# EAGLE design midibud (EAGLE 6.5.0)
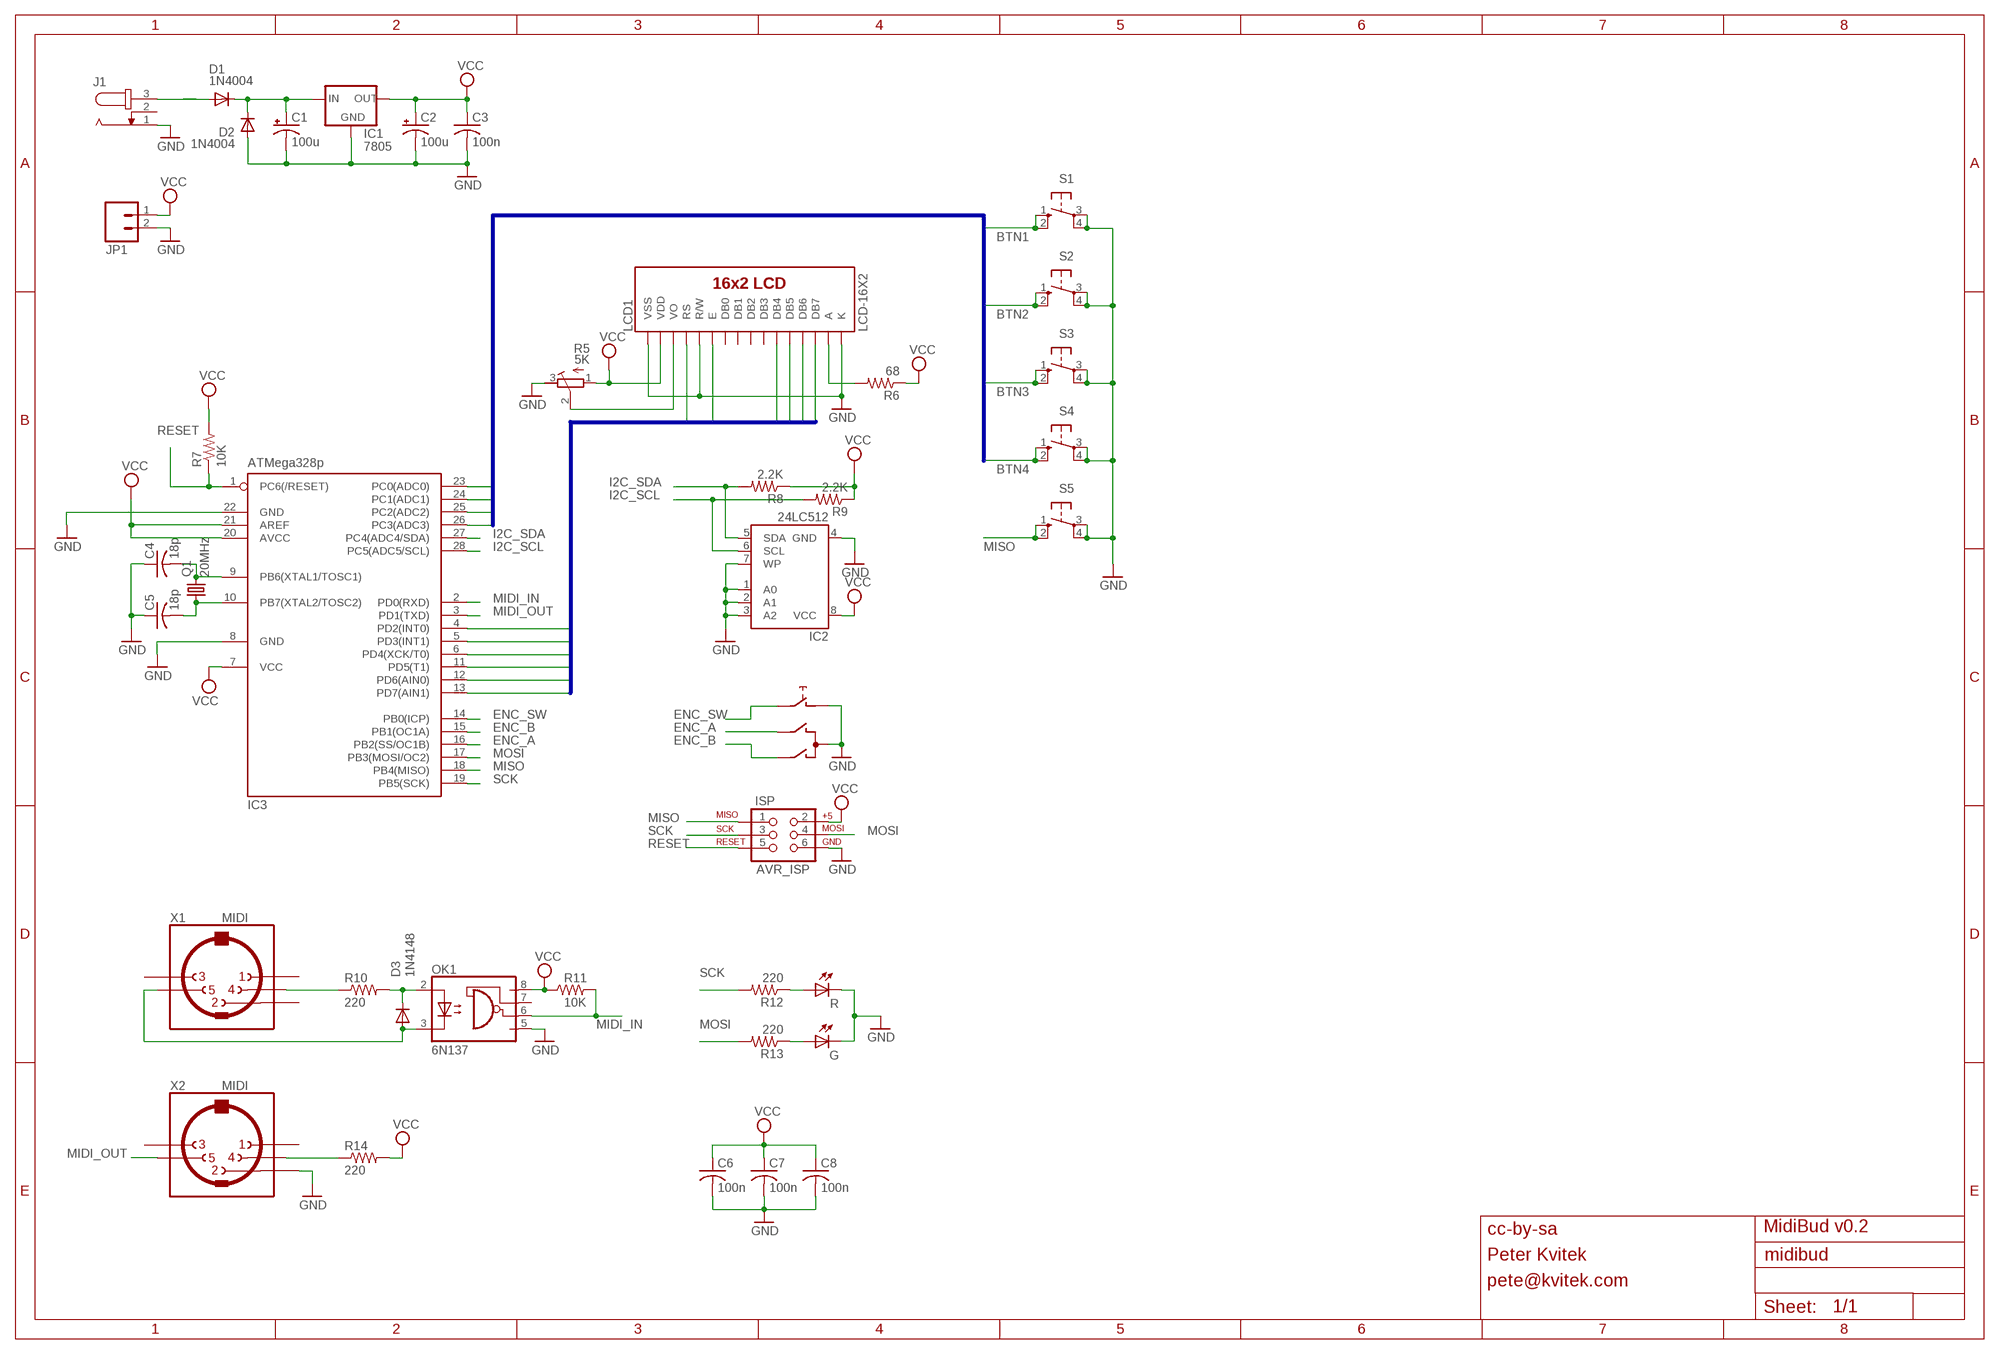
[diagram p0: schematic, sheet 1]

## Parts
C1  100u  CPOL-USE2.5-7  [E2,5-7]
C2  100u  CPOL-USE2.5-7  [E2,5-7]
C3  100n  C-US025-025X050  [C025-025X050]
C4  18p  C-US025-024X044  [C025-024X044]
C5  18p  C-US025-024X044  [C025-024X044]
C6  100n  C-US025-025X050  [C025-025X050]
C7  100n  C-US025-025X050  [C025-025X050]
C8  100n  C-US025-025X050  [C025-025X050]
D1  1N4004  [DO41-10]
D2  1N4004  [DO41-10]
D3  1N4148  DIODE-D-5  [D-5]
ENC1  Encoder  EC12E_SW  [ALPS_EC12E_SW]
G  LED3MM  [LED3MM]
IC1  7805  V_REG_78XXSIDE  [78XXL]
IC2  24LC512  AT24CP  [DIL08]
IC3  ATMega328p  MEGA8-P  [DIL28-3]
ISP  AVR_ISP  AVR_SPI_PRG_6PTH  [2X3]
J1  JACK-PLUG  [SPC4078_LARGER_HOLES]
JP1  M02  [1X02_LONGPADS]
LCD1  LCD-16X2  [LCD-16X2]
OK1  6N137  [DIL08]
Q1  20MHz  CRYSTALHC49U-V  [HC49U-V]
R  LED3MM  [LED3MM]
R5  5K  R-TRIMM3296P  [RTRIM3296P]
R6  68  R-US_0204/7  [0204/7]
R7  10K  R-US_0204/7  [0204/7]
R8  2.2K  R-US_0204/7  [0204/7]
R9  2.2K  R-US_0204/7  [0204/7]
R10  220  R-US_0204/7  [0204/7]
R11  10K  R-US_0204/7  [0204/7]
R12  220  R-US_0204/7  [0204/7]
R13  220  R-US_0204/7  [0204/7]
R14  220  R-US_0204/7  [0204/7]
S1  40-XX  [B3F-40XX]
S2  40-XX  [B3F-40XX]
S3  40-XX  [B3F-40XX]
S4  40-XX  [B3F-40XX]
S5  40-XX  [B3F-40XX]
X1  MIDI  MAB5SH  [MAB5SH]
X2  MIDI  MAB5SH  [MAB5SH]

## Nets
BTN1: IC3.23(PC0(ADC0)) S1.1(S) S1.2(S1)
BTN2: IC3.24(PC1(ADC1)) S2.1(S) S2.2(S1)
BTN3: IC3.25(PC2(ADC2)) S3.1(S) S3.2(S1)
BTN4: IC3.26(PC3(ADC3)) S4.1(S) S4.2(S1)
ENC_A: ENC1.B IC3.16(PB2(SS/OC1B))
ENC_B: ENC1.A IC3.15(PB1(OC1A))
ENC_SW: ENC1.E IC3.14(PB0(ICP))
GND: C1.- C2.- C3.2 C4.1 C5.1 C6.2 C7.2 C8.2 D2.A ENC1.C ENC1.D G.K(C) IC1.GND IC2.1(A0) IC2.2(A1) IC2.3(A2) IC2.4(GND) IC2.7(WP) IC3.8(GND) IC3.22(GND) ISP.6 J1.1 JP1.2 LCD1.1(VSS) LCD1.5(R/W) LCD1.16(K) OK1.5(GND) R5.3(E) R.K(C) S1.3(P) S1.4(P1) S2.3(P) S2.4(P1) S3.3(P) S3.4(P1) S4.3(P) S4.4(P1) S5.3(P) S5.4(P1) X2.2
I2C_SCL: IC2.6(SCL) IC3.28(PC5(ADC5/SCL)) R9.2
I2C_SDA: IC2.5(SDA) IC3.27(PC4(ADC4/SDA)) R8.2
LCD_DATA1: IC3.6(PD4(XCK/T0)) LCD1.11(DB4)
LCD_DATA2: IC3.11(PD5(T1)) LCD1.12(DB5)
LCD_DATA3: IC3.12(PD6(AIN0)) LCD1.13(DB6)
LCD_DATA4: IC3.13(PD7(AIN1)) LCD1.14(DB7)
LCD_EN: IC3.5(PD3(INT1)) LCD1.6(E)
LCD_RS: IC3.4(PD2(INT0)) LCD1.4(RS)
MIDI_IN: IC3.2(PD0(RXD)) OK1.6(VO) R11.2
MIDI_OUT: IC3.3(PD1(TXD)) X2.5
MISO: IC3.18(PB4(MISO)) ISP.1 S5.1(S) S5.2(S1)
MOSI: IC3.17(PB3(MOSI/OC2)) ISP.4 R13.2
N$2: D3.C OK1.2(A) R10.2
N$3: R14.1 X2.4
N$25: R12.1 R.A
N$26: G.A R13.1
N$72: R10.1 X1.4
N$73: D3.A OK1.3(C) X1.5
N$78: LCD1.3(VO) R5.2(S)
N$79: LCD1.15(A) R6.2
N$82: C5.2 IC3.10(PB7(XTAL2/TOSC2)) Q1.1
N$83: C4.2 IC3.9(PB6(XTAL1/TOSC1)) Q1.2
RESET: IC3.1(PC6(/RESET)) ISP.5 R7.1
SCK: IC3.19(PB5(SCK)) ISP.3 R12.2
VCC: C2.+ C3.1 C6.1 C7.1 C8.1 IC1.OUT IC2.8(VCC) IC3.7(VCC) IC3.20(AVCC) IC3.21(AREF) ISP.2 JP1.1 LCD1.2(VDD) OK1.8(VCC) R5.1(A) R6.1 R7.2 R8.1 R9.1 R11.1 R14.2
VPWR: D1.A J1.3
VREGIN: C1.+ D1.C D2.C IC1.IN
Unconnected: ENC1.GND1(G) ENC1.GND2(G) J1.2 LCD1.7(DB0) LCD1.8(DB1) LCD1.9(DB2) LCD1.10(DB3) OK1.7(VE) X1.1 X1.2 X1.3 X2.1 X2.3

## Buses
LCD_RS,LCD_EN,LCD_DATA[1..4]
BTN[1..4]

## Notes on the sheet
- cc-by-sa | MidiBud v0.2
- Peter Kvitek
- pete@kvitek.com

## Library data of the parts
C1 C2 = rcl:CPOL-US: POLARIZED CAPACITOR, American symbol
C3-C8 = rcl:C-US: CAPACITOR, American symbol
D1 D2 = diode:1N4004: DIODE
D3 = diode:DIODE-: DIODE
ENC1 = switch-alps:EC12E_SW: ALPS rotary Encoder EC12E series with switch
G R = led:LED: LED
IC1 = SparkFun:V_REG_78XX: Voltage Regulator Standard 7805 5V regulator. IGO (Input Ground Output). Spark Fun Electronics SKU : COM-00107
IC2 = atmel:AT24C*: 2-wire serial EEPROM
IC3 = atmel:MEGA8-P: MICROCONTROLLER 8 Kbytes FLASH, 1 kbytes SRAM, 512 bytes EEPROM, USART, 4-channel 10 bit ADC, 2-channel 8 bit ADC Pin compatible with Atmega48, ATMega88, ATMega168 Source: avr.lbr; OC_FARNELL: unknown; OC_NEWARK: unknown
ISP = SparkFun:AVR_SPI_PRG_6: AVR ISP 6 Pin This is the reduced ISP connector for AVR programming. Common on Arduino. This footprint will take up less PCB space and can be used with a 10-pin to 6-pin adapter such as SKU: BOB-08508
J1 = con-jack2:JACK-PLUG: DC POWER JACK Power Jack, DC, Right Angle, Through Hole, Rated 5A at 16VDC, PC Terminals Distributor: Farnell (www.Farnell.de) Drawing: 84N1161.pdf / 84N1162.pdf Manufacturer: SPC Technology (www.spctechnology.com) Type: SPC4077 / SPC 4078
JP1 = SparkFun:M02: Header 2
LCD1 = SparkFun:LCD-16X2
OK1 = kvitekp:6N137: MOTOROLA OPTO COUPLER; MPN: 6N137; OC_FARNELL: 1328376; OC_NEWARK: 52M1895
Q1 = crystal:CRYSTAL: CRYSTAL; OC_FARNELL: 1666969; OC_NEWARK: unknown
R5 = rcl:R-TRIMM: Trimm resistor
R6-R14 = rcl:R-US_: RESISTOR, American symbol
S1-S5 = og-switch:40-XX: OMRON SWITCH
X1 X2 = og-midi:MAB5SH: Female CONNECTOR 5 pins 90 deg. with shield, horizontal (DIN 41524)

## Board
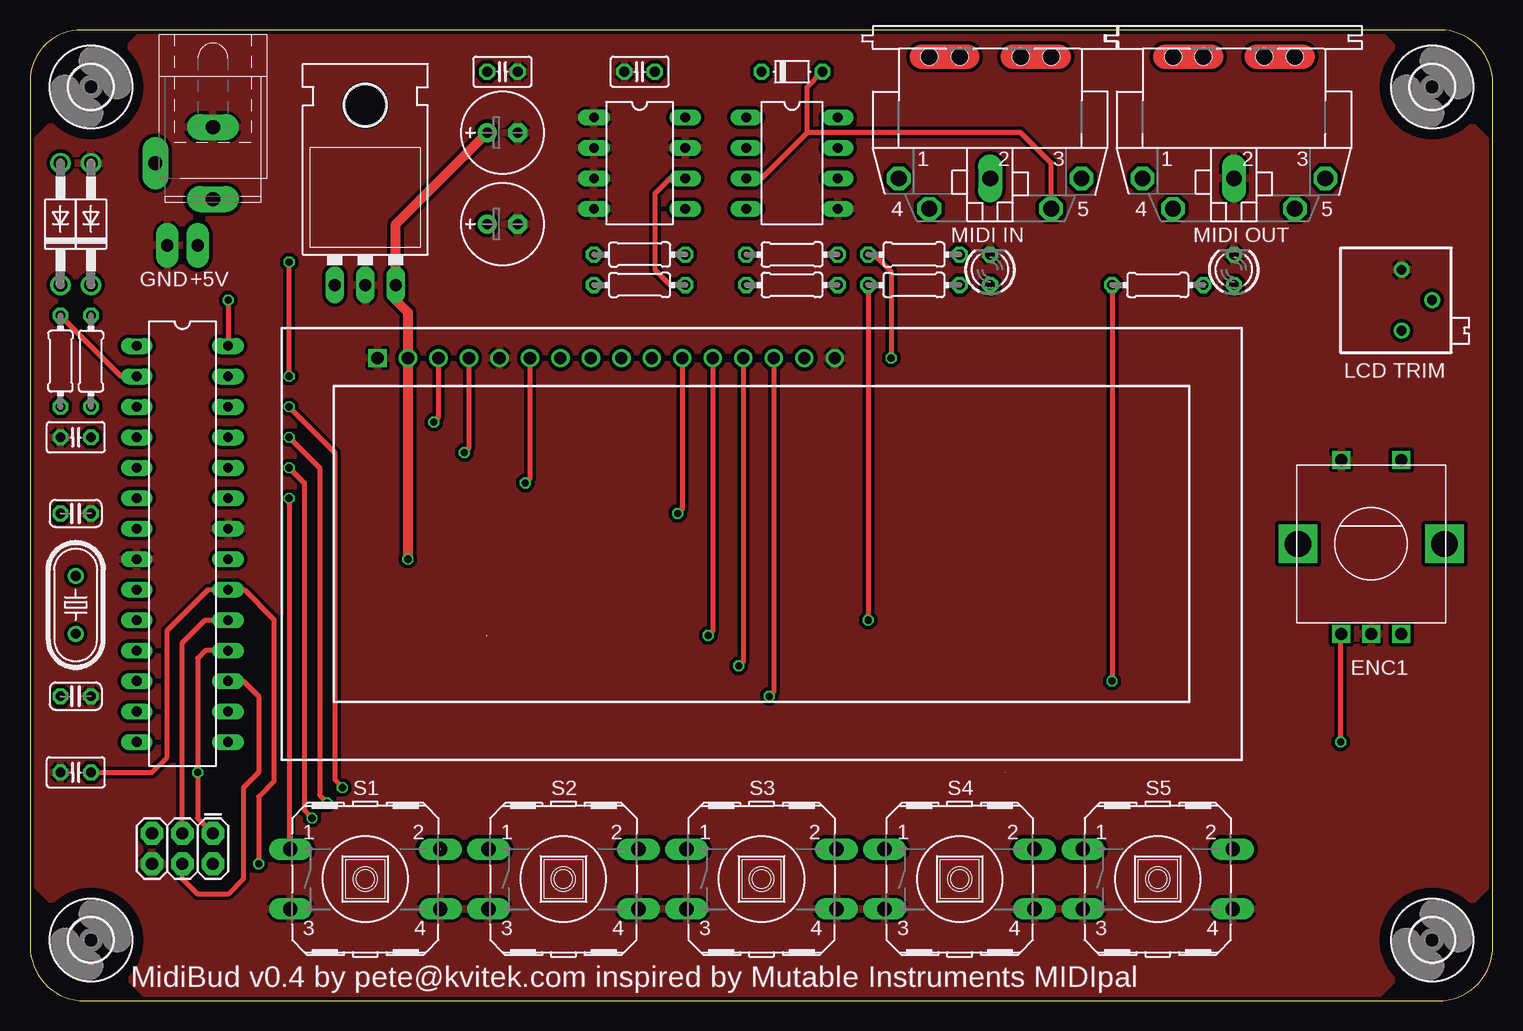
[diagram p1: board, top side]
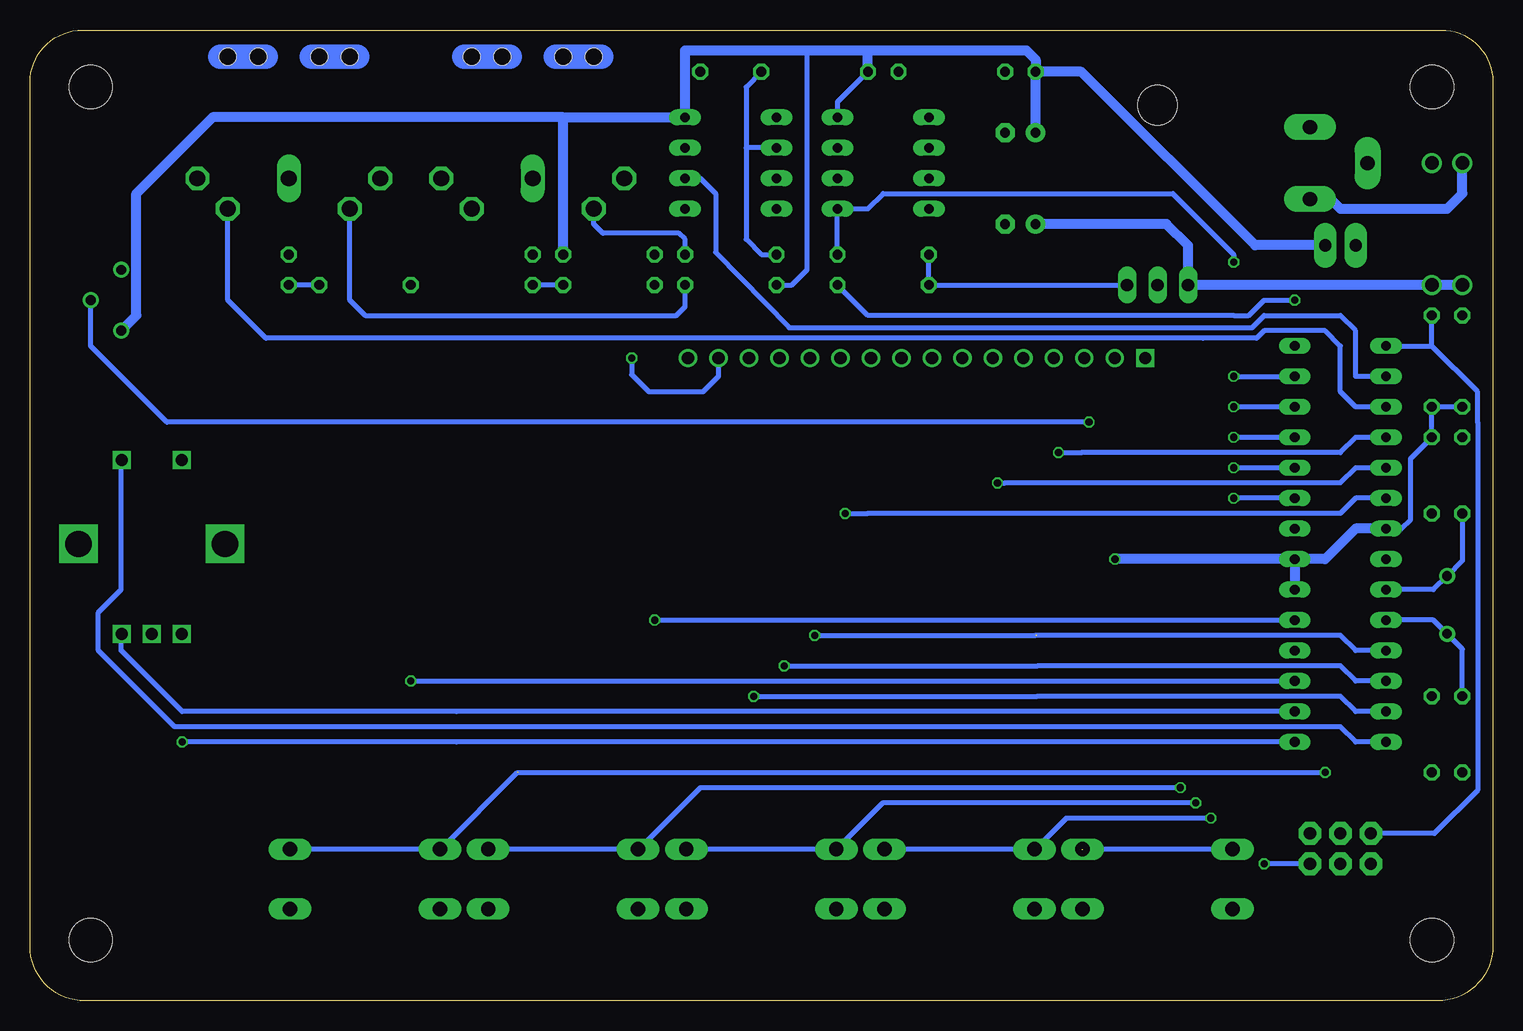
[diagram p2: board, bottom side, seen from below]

Size 121.9 x 80.95 mm. Coordinates in mm from the lower left corner, seen from the top.
Outline: 4.58,0 117.34,0 arc90 121.9,4.56 121.9,76.56 arc90 117.51,80.95 4.31,80.95 arc90 0,76.64 0,4.58 arc90 4.58,0
Copper layers (1*16): Top 0.035mm / dielectric 1.5mm / Bottom 0.035mm
Design rules "default": minimum track width 8mil, minimum drill 16mil, track to track 8mil, track to pad 8mil, pad to pad 8mil, via to via 8mil, smd to smd 0mil, copper to edge 10mil, drill to drill 10mil, minimum pad ring 10mil, minimum via ring 6mil, stop-mask expansion 2mil, vias tented up to drill 100mil, thermal gap 10mil

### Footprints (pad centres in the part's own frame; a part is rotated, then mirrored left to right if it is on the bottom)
E2,5-7 = drill 0.813 pad 1.6: + -1.27,0 | drill 0.813 pad 1.6 octagon: - 1.27,0
C025-025X050 = drill 0.813 octagon: 1 -1.27,0; 2 1.27,0
C025-024X044 = drill 0.813 octagon: 1 -1.27,0; 2 1.27,0
DO41-10 = drill 1.118: A 5.08,0; C -5.08,0
D-5 = drill 0.813 octagon: A 2.54,0; C -2.54,0
ALPS_EC12E_SW = drill 1 square: A -2.5,-7.5; B 2.5,-7.5; C 0,-7.5; D -2.5,7; E 2.5,7 | drill 2.2 square: GND1 -6.1,0; GND2 6.1,0
LED3MM = drill 0.813 octagon: A -1.27,0; K 1.27,0
78XXL = drill 1.016 long: GND 0,-3.81; IN -2.54,-3.81; OUT 2.54,-3.81 | hole 3.302: 0,11.176
DIL08 = drill 0.813 long: 1 -3.81,-3.81; 2 -1.27,-3.81; 3 1.27,-3.81; 4 3.81,-3.81; 5 3.81,3.81; 6 1.27,3.81; 7 -1.27,3.81; 8 -3.81,3.81
DIL28-3 = drill 0.813 long: 1 -16.51,-3.81; 2 -13.97,-3.81; 3 -11.43,-3.81; 4 -8.89,-3.81; 5 -6.35,-3.81; 6 -3.81,-3.81; 7 -1.27,-3.81; 8 1.27,-3.81; 9 3.81,-3.81; 10 6.35,-3.81; 11 8.89,-3.81; 12 11.43,-3.81; 13 13.97,-3.81; 14 16.51,-3.81; 15 16.51,3.81; 16 13.97,3.81; 17 11.43,3.81; 18 8.89,3.81; 19 6.35,3.81; 20 3.81,3.81; 21 1.27,3.81; 22 -1.27,3.81; 23 -3.81,3.81; 24 -6.35,3.81; 25 -8.89,3.81; 26 -11.43,3.81; 27 -13.97,3.81; 28 -16.51,3.81
2X3 = drill 1.016 pad 1.88 octagon: 1 0,0; 2 0,2.54; 3 2.54,0; 4 2.54,2.54; 5 5.08,0; 6 5.08,2.54
SPC4078_LARGER_HOLES = drill 1.2 pad 2.184 long: 1 -3,0; 2 0,-4.8; 3 3,0
1X02_LONGPADS = drill 1.016 pad 1.88 long: 1 0,0; 2 2.54,0
LCD-16X2 = drill 1.016 square: 1 -32,15.5 | drill 1.016: 2 -29.46,15.5; 3 -26.92,15.5; 4 -24.38,15.5; 5 -21.84,15.5; 6 -19.3,15.5; 7 -16.76,15.5; 8 -14.22,15.5; 9 -11.68,15.5; 10 -9.14,15.5; 11 -6.6,15.5; 12 -4.06,15.5; 13 -1.52,15.5; 14 1.02,15.5; 15 3.56,15.5; 16 6.1,15.5
HC49U-V = drill 0.813: 1 -2.413,0; 2 2.413,0
RTRIM3296P = drill 0.813: 1 0,-2.54; 2 2.54,0; 3 0,2.54
0204/7 = drill 0.813 octagon: 1 -3.81,0; 2 3.81,0
B3F-40XX = drill 1.194 long: 1 -6.248,2.489; 2 6.248,2.489; 3 -6.248,-2.489; 4 6.248,-2.489
3,6 = hole 3.6: 0,0
MAB5SH = drill 1.321 octagon: 1 7.62,7.62; 3 -7.62,7.62; 4 5.08,10.16; 5 -5.08,10.16 | drill 1.321 long: 2 0,7.62 | hole 1.4: 2.54,-2.54; -2.54,-2.54; -5.08,-2.54; 5.08,-2.54

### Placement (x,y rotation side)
C1  39.37,64.77 0 top
C2  39.37,72.39 0 top
C3  50.8,77.47 180 top
C4  3.81,40.64 180 top
C5  3.81,25.4 180 top
C6  3.81,46.99 180 top
C7  3.81,19.05 180 top
C8  39.37,77.47 0 top
D1  2.54,64.77 90 top
D2  5.08,64.77 90 top
D3  63.5,77.47 0 top
ENC1  111.76,38.1 0 top
G  100.33,60.96 90 top
IC1  27.94,63.5 0 top
IC2  50.8,69.85 270 top
IC3  12.7,38.1 270 top
ISP  15.24,13.97 180 top
J1  15.24,69.85 270 top
JP1  13.97,62.99 180 top
LCD1  60.96,38.1 0 top
OK1  63.5,69.85 270 top
Q1  3.81,33.02 90 top
R  80.01,60.96 90 top
R5  114.3,58.42 0 top
R6  73.66,62.23 180 top
R7  5.08,53.34 270 top
R8  50.8,62.23 0 top
R9  50.8,59.69 0 top
R10  63.5,62.23 180 top
R11  2.54,53.34 90 top
R12  73.66,59.69 180 top
R13  93.98,59.69 180 top
R14  63.5,59.69 180 top
S1  27.94,10.16 0 top
S2  44.45,10.16 0 top
S3  60.96,10.16 0 top
S4  77.47,10.16 0 top
S5  93.98,10.16 0 top
U$2  [3,6]  5.08,5.08 0 top
U$3  [3,6]  5.08,76.2 0 top
U$4  [3,6]  116.84,76.2 0 top
U$5  [3,6]  116.84,5.08 0 top
X1  80.01,76.2 180 top
X2  100.33,76.2 180 top

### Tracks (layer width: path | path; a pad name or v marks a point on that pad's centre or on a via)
BTN1  (via drill 0.6)  (1 unrouted)
  Top 0.406: v21.59,41.91 21.59,12.75 S1.1
  Bottom 0.406: S1.1 34.24,12.65 | IC3.23 v21.59,41.91
BTN2  (via drill 0.6)
  Top 0.406: v21.59,44.45 22.86,43.18 22.86,15.88 v23.5,15.24
  Bottom 0.406: S2.2 S2.1 38.15,12.65 38.1,12.7 35.56,15.24 v23.5,15.24 | IC3.24 v21.59,44.45
BTN3  (via drill 0.6)
  Top 0.406: v21.59,46.99 24.13,44.45 24.13,17.14 v24.77,16.51
  Bottom 0.406: S3.2 S3.1 50.85,16.51 v24.77,16.51 | IC3.25 v21.59,46.99
BTN4  (via drill 0.6)
  Top 0.406: v21.59,49.53 25.4,45.72 25.4,18.41 v26.04,17.78
  Bottom 0.406: S4.2 S4.1 71.17,12.65 71.12,12.7 66.04,17.78 v26.04,17.78 | IC3.26 v21.59,49.53
ENC_A
  Bottom 0.406: IC3.16 86.36,24.13 109.22,24.13 114.3,29.21 114.3,30.56 ENC1.B
ENC_B  (via drill 0.6)
  Top 0.406: v109.22,21.59 109.22,30.56 ENC1.A
  Bottom 0.406: IC3.15 86.36,21.59 v109.22,21.59
ENC_SW
  Bottom 0.406: IC3.14 11.43,21.59 12.7,22.86 86.36,22.86 102.87,22.86 109.86,22.86 116.2,29.21 116.2,32.38 114.3,34.29 114.3,45.06 ENC1.E
GND
  pour Top (isolate 0.305): 0,10.2 0,71.23 9.49,80.72 112.35,80.72 121.62,71.45 121.62,9.81 112.16,0.36 9.84,0.36
I2C_SCL  (via drill 0.6)
  Top 0.406: v16.51,58.42 IC3.28 | IC2.6 53.34,68.58 52.07,67.31 52.07,60.96 53.34,59.69 R9.2
  Bottom 0.406: R9.2 52.07,57.15 21.59,57.15 20.32,57.15 19.05,58.42 v16.51,58.42
I2C_SDA  (via drill 0.6, 0.61)
  Top 0.406: v21.59,52.07 v21.59,61.59
  Bottom 0.406: R8.2 IC2.5 52.07,66.04 50.8,67.31 26.67,67.31 21.59,62.23 v21.59,61.59 | v21.59,52.07 IC3.27
LCD_DATA1  (via drill 0.6)
  Top 0.406: LCD1.11 54.36,41.02 v53.98,40.64
  Bottom 0.406: IC3.6 11.43,41.91 12.7,40.64 52.07,40.64 v53.98,40.64
LCD_DATA2  (via drill 0.6)  (1 unrouted)
  Top 0.406: LCD1.12 56.9,30.86 v56.52,30.48
  Bottom 0.406: IC3.11 11.43,29.21 12.7,30.48 38.02,30.48 | v56.52,30.48 38.1,30.48
LCD_DATA3  (via drill 0.6)
  Top 0.406: LCD1.13 59.44,28.32 v59.05,27.94
  Bottom 0.406: IC3.12 11.43,26.67 12.7,27.94 37.91,27.94 v59.05,27.94
LCD_DATA4  (via drill 0.6)
  Top 0.406: LCD1.14 61.98,25.79 v61.59,25.4
  Bottom 0.406: IC3.13 11.43,24.13 12.7,25.4 37.95,25.4 v61.59,25.4
LCD_EN  (via drill 0.6)
  Top 0.406: LCD1.6 41.66,43.56 v41.27,43.18
  Bottom 0.406: IC3.5 11.43,44.45 12.7,43.18 40.64,43.18 v41.27,43.18
LCD_RS  (via drill 0.6)
  Top 0.406: LCD1.4 36.58,46.1 v36.2,45.72
  Bottom 0.406: IC3.4 11.43,46.99 12.7,45.72 34.29,45.72 v36.2,45.72
MIDI_IN
  Top 0.406: IC3.2 7.62,52.07 R11.2
  Bottom 0.406: OK1.6 66.04,68.58 64.77,67.31 64.77,62.39 58.64,56.13 20.07,56.13 19.05,57.15 12.7,57.15 11.43,55.88 11.43,52.07 IC3.2
MIDI_OUT
  Bottom 0.406: X2.5 105.41,58.42 102.23,55.24 24.13,55.24 19.68,55.24 19.05,55.88 13.97,55.88 12.7,54.61 12.7,50.8 11.43,49.53 IC3.3
MISO  (via drill 0.6)  (1 unrouted)
  Top 0.406: IC3.18 14.61,29.21 13.97,28.57 v13.97,19.05 13.97,15.24 ISP.1
  Bottom 0.406: S5.2 S5.1 87.68,12.65 87.63,12.7 81.28,19.05 | 81.23,19.05 30.23,19.05 19.05,19.05 v13.97,19.05
MOSI  (via drill 0.6)
  Top 0.406: R13.2 v90.17,26.67 | IC3.17 17.78,26.67 19.05,25.4 19.05,19.05 17.78,17.78 17.78,10.16 16.51,8.89 13.97,8.89 12.7,10.16 ISP.4
  Bottom 0.406: v90.17,26.67 IC3.17
N$2
  Bottom 0.406: D3.C 62.23,76.2 62.23,71.12 | 62.23,71.12 62.23,63.5 60.96,62.23 R10.2 | OK1.2 62.23,71.12
N$3
  Bottom 0.406: R14.1 67.31,57.87 68.03,57.15 93.98,57.15 95.25,58.42 X2.4
N$25
  Bottom 0.406: R12.1 R.A
N$26
  Bottom 0.406: R13.1 G.A
N$72
  Bottom 0.406: R10.1 67.31,63.5 67.82,64.01 74.17,64.01 74.93,64.77 X1.4
N$73
  Top 0.406: 64.77,72.39 64.77,76.2 D3.A | X1.5 85.09,69.85 82.55,72.39 64.77,72.39 | OK1.3 60.96,68.58 64.77,72.39
N$78  (via drill 0.6)
  Top 0.406: LCD1.3 34.04,48.65 v33.66,48.26
  Bottom 0.406: v33.66,48.26 110.49,48.26 116.84,54.61 R5.2
N$79  (via drill 0.61)
  Top 0.406: R6.2 70.33,62.23 71.75,60.81 v71.75,53.59
  Bottom 0.406: v71.75,53.59 71.75,52.22 70.33,50.8 65.81,50.8 64.52,52.09 LCD1.15
N$82
  Bottom 0.406: IC3.10 4.95,31.75 Q1.1 2.54,29.34 C5.2
N$83
  Bottom 0.406: IC3.9 4.95,34.29 Q1.2 2.54,36.7 C4.2
RESET
  Bottom 0.406: ISP.5 4.86,13.97 1.27,17.56 1.27,48.26 1.27,50.8 5.08,54.61 | 5.08,54.61 R7.1 | IC3.1 5.08,54.61
SCK  (via drill 0.6)
  Top 0.406: ISP.3 12.7,29.84 14.61,31.75 IC3.19 | R12.2 v69.85,31.75
  Bottom 0.406: v69.85,31.75 IC3.19
VCC  (via drill 0.6, 0.61)
  Top 0.406: v19.05,11.43 19.05,17.02 20.32,18.29 20.32,31.82 17.85,34.29 IC3.20 14.85,34.29 11.43,30.87 11.43,20.32 10.16,19.05 C7.1
  Top 0.813: v31.5,36.83 LCD1.2 31.5,57.4 30.48,58.42 IC1.OUT 30.48,64.77 C2.+
  Bottom 0.406: IC3.7 7.62,39.37 6.86,40.13 6.86,45.21 C6.1 R7.2 R11.1 | C3.1 54.61,74.93 IC2.8 | IC1.OUT R9.1 R8.1 | ISP.2 v19.05,11.43 | R14.2 58.42,59.69 57.15,60.96 57.15,79.25
  Bottom 0.813: IC3.21 v31.5,36.83 | IC3.7 11.43,39.37 13.97,36.83 IC3.21 | C2.+ C8.1 | 52.07,79.25 57.15,79.25 67.31,79.25 OK1.8 77.47,73.66 | 52.07,79.25 38.86,79.25 38.1,78.49 C8.1 | C3.1 52.07,79.25 | IC3.21 IC3.20 | R6.1 77.47,73.66 | 77.47,73.66 106.68,73.66 113.03,67.31 113.03,57.15 R5.1 | JP1.1 19.81,62.99 34.29,77.47 C8.1
VPWR
  Bottom 0.813: J1.3 13.51,66.85 12.7,66.04 3.81,66.04 2.54,67.31 D1.A
VREGIN
  Bottom 0.813: D1.C D2.C IC1.IN 25.4,62.97 27.2,64.77 C1.+

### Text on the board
tNames: MIDI IN | MIDI OUT | GND | +5V | LCD TRIM | MidiBud v0.4 by pete@kvitek.com inspired by Mutable Instruments MIDIpal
